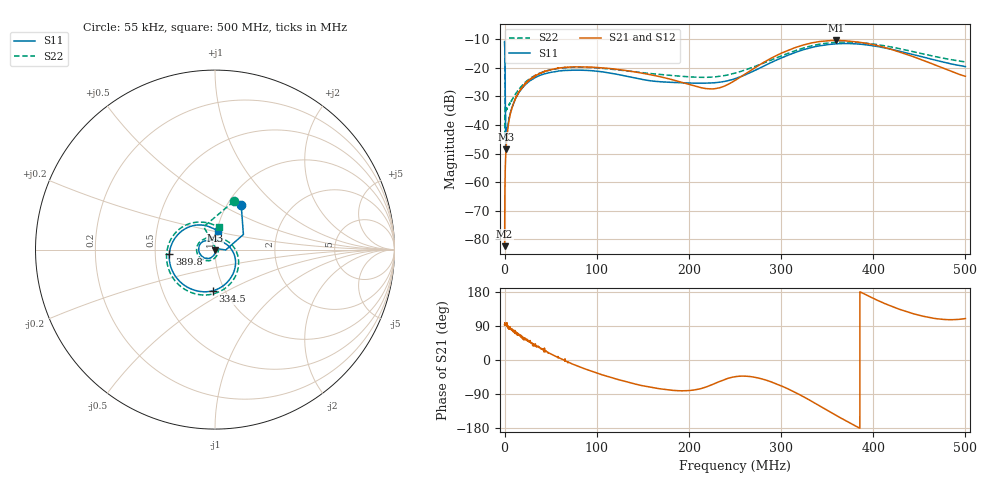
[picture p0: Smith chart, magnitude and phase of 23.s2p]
#  HZ  S  MA  R  50.00
! Rohde & Schwarz Vector Network Analyzer
! Rohde-Schwarz,ZNL6-2Port,1323001206101378,1.50.1.34-21.10.1.104
! Created: UTC 10/21/2024, 2:42:00 AM
! freq[Hz]  mag:S11  ang:S11  mag:S21  ang:S21  mag:S12  ang:S12  mag:S22  ang:S22
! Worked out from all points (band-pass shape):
!   10000 points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, 55 kHz to 500 MHz, reference 50 ohm
!   highest |S21| = -10.42 dB at 359.7 MHz (marker M1); lowest = -82.4 dB at 55 kHz (marker M2)
!   |S21| within 3 dB of the highest: 311.1 MHz to 418.4 MHz (107.3 MHz wide, 29.4 % of centre)
!   lowest |S11| = -48.6 dB at 1.255 MHz (marker M3), VSWR 1.01, Z = 49.9 - j0.365 ohm
!   |S11| at or under -10 dB: start of sweep to end of sweep
!   |S22| runs from -44.5 to -10.8 dB; largest |S21 - S12| = 0.019
!   S11 on the Smith chart (normalised r, x): 55 kHz: 1.16, +0.63; 334.5 MHz: 0.88, -0.43; 389.8 MHz: 0.59, -0.03; 500 MHz: 1.01, +0.21
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54999.5  0.2882 59.6  7.613e-05 93.0  6.583e-05 85.7  0.2879 68.8
1254988  0.003736 -102.1  0.002884 93.4  0.002897 93.6  0.0203 -11.9
2654974  0.009045 -61.0  0.006826 96.0  0.005888 82.7  0.01909 -26.8
3254968  0.009126 -68.6  0.007925 86.8  0.007799 89.2  0.02048 -27.5
3654964  0.01027 -72.0  0.009062 88.9  0.008693 84.9  0.02081 -31.3
5004950  0.0132 -81.0  0.01247 85.0  0.01207 83.3  0.0228 -40.1
9754902  0.02367 -95.3  0.024 76.2  0.02394 75.6  0.03066 -65.7
1.785482e7  0.04155 -109.4  0.04236 61.2  0.04349 64.7  0.04697 -91.1
2.97547e7  0.06282 -127.4  0.06704 44.9  0.0662 44.3  0.06859 -116.4
4.255457e7  0.07792 -147.1  0.08515 25.7  0.08519 25.5  0.08555 -136.8
8.340417e7  0.09093 168.9  0.1043 -19.9  0.1044 -19.9  0.1027 177.3
1.667033e8  0.05752 113.5  0.07107 -75.3  0.07125 -75.4  0.07721 120.9
2.220528e8  0.05425 72.2  0.04286 -68.2  0.0428 -68.0  0.06857 76.3
2.500525e8  0.06461 34.9  0.06025 -44.0  0.06018 -43.5  0.08076 38.9
3.00452e8  0.1491 -41.1  0.1808 -68.5  0.1806 -67.2  0.1619 -36.4
3.333517e8  0.2281 -91.4  0.2731 -109.0  0.2738 -107.2  0.2432 -89.4
3.344517e8  0.2302 -93.1  0.2755 -110.5  0.276 -108.8  0.2455 -91.2
3.596514e8  0.2626 -132.2  0.3012 -146.0  0.3013 -144.0  0.2796 -130.2
3.897511e8  0.2557 -174.5  0.273 174.8  0.2744 176.4  0.2721 -172.8
4.167008e8  0.216 153.2  0.2172 144.7  0.217 145.8  0.236 154.7
4.571504e8  0.1501 115.3  0.1298 113.9  0.13 114.4  0.1707 116.1
5e8  0.1051 81.6  0.0712 109.4  0.07117 109.6  0.1269 80.8
